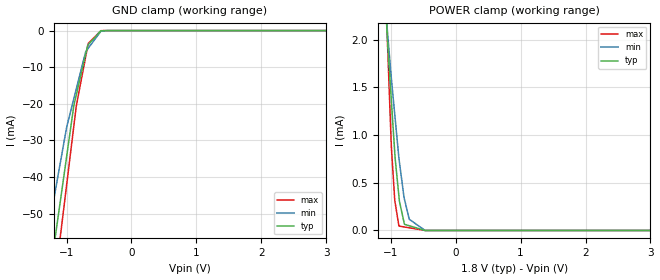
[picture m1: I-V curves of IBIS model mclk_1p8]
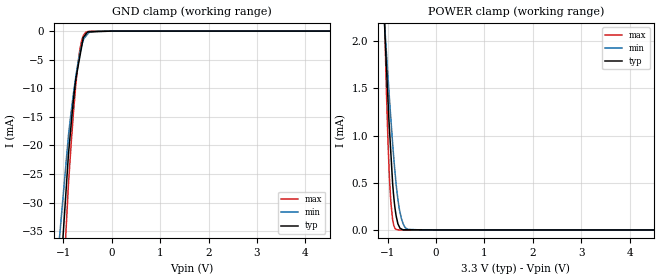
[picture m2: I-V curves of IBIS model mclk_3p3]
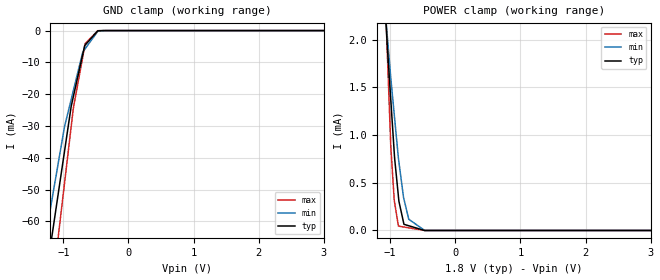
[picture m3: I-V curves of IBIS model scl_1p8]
|Texas Instruments Incorporated
| Low-Power Stereo Codec with 6 Inputs, 6 Outputs, Speaker/HP Amp and
| Enhanced Digital Effects
| Marketing part#   Digital Voltage Range   Package-type   #pins
| TLV320AIC3101IRHBR   1.1V - 3.6V   QFN   32
| TLV320AIC3101IRHBT   1.1V - 3.6V   QFN   32
| TLVAIC3101IRHBRG4   1.1V - 3.6V   QFN   32
| TLVAIC3101IRHBTG4   1.1V - 3.6V   QFN   32
[IBIS Ver]   4.1
[File name]   tlv320aic3101.ibs
[File Rev]   1.1
[Date]   10/26/2012
[Source]
| Texas Instruments Incorporated.
| Analog-eLab Design Center, HPA
| 12500 TI Blvd
| Dallas, TX -75243
| e-mail: elab_scm_ibis@list.ti.com
[Notes]   Revision History:
| Rev 1.1: 10/26/2012
| - Voltage range for modeling is changed for 3.3V models.
| Rev 1.0: 10/23/2012
| - Initial version of the model
| - Model generated from simulations in TISPICE
| - Model matched to SPICE simulation
| - C_comp although listed in numerical order of value are
|   obtained from varying PVT conditions. For PVT conditions for
|   each specific value refer the buffer description under
|   respective [Model]. IBIS model user is responsible for using
|   appropriate C_comp to simulate for Signal Integrity.
| - Model names with a trailing _1p8 contains the model for
|   1.8V [1.71V and 1.89V].Model names with a trailing _3p3
|   contains the model for 3.3V [2.7V and 3.6V].
| - The buffer characteristics for buffer on Pins (MCLK),
|   (DIN) and (_RESET) is same, hence replaced by a single model "mclk".
[Disclaimer]
| This model is designed as an aid for customers of Texas Instruments.
| TI and its licensors and suppliers make no warranties, either expressed
| or implied, with respect to this  model, including the warranties of
| merchantability or fitness for a particular purpose. The model is
| provided solely on an "as is" basis. The entire risk as to its quality
| and performance is with the customer.
[Copyright]
(C) Copyright 2012 Texas Instruments Incorporated.All rights reserved.
|   TLV320AIC3101
[Component]   TLV320AIC3101
[Manufacturer]   TI
[Package]   |32 QFN   -  RHB package
|   typ   min   max
R_pkg   0.07718   0.03258   0.11084
L_pkg   1.34741nH   0.76736nH   1.81874nH
C_pkg   0.19486pF   0.16263pF   0.25079pF
[Pin]  signal_name   model_name   R_pin   L_pin   C_pin
1   MCLK   MCLK   0.10980   1.80738nH  0.20351pF
2   BCLK   BW_CLK   0.04834   1.27894nH  0.25079pF
3   WCLK   BW_CLK   0.04153   1.05595nH  0.22423pF
4   DIN   MCLK   0.07341   1.17495nH  0.17505pF
5   DOUT   DOUT   0.06543   1.04328nH  0.16455pF
6   DVSS   GND   0.06617   1.05558nH  0.16473pF
7   IOVDD   POWER   0.07422   1.18976nH  0.17262pF
8   SCL   SCL   0.09445   1.54209nH  0.17632pF
9   SDA   SDA   0.10381   1.70349nH  0.18628pF
10   MIC1LP/LINE1LP   TERM   0.09706   1.57875nH  0.19190pF
11   MIC1LM/LINE1LM   TERM   0.11084   1.81874nH  0.21129pF
12   MIC1RP/LINE1RP   TERM   0.09921   1.61505nH  0.20474pF
13   MIC1RM/LINE1RM   TERM   0.09378   1.51996nH  0.19828pF
14   MIC2L/LINE2L/MICDET TERM   0.09457   1.53226nH  0.19911pF
15   MICBIAS   TERM   0.10123   1.64737nH  0.20366pF
16   MIC2R/LINE2R   TERM   0.11073   1.81870nH  0.19581pF
17   AVSS1   GND   0.10587   1.73309nH  0.18653pF
18   DRVDD   POWER   0.08549   1.37555nH  0.18063pF
19   HPLOUT   TERM   0.04394   1.15760nH  0.22090pF
20   HPLCOM   TERM   0.03761   0.93514nH  0.20874pF
21   DRVSS   GND   0.03475   0.83845nH  0.19402pF
22   HPRCOM   TERM   0.03258   0.76736nH  0.18547pF
23   HPROUT   TERM   0.03636   0.90542nH  0.19865pF
24   DRVDD   POWER   0.04412   1.17412nH  0.20375pF
25   AVDD   POWER   0.04645   1.25584nH  0.20175pF
26   AVSS2   GND   0.04847   1.29980nH  0.22244pF
27   LEFT_LOP   TERM   0.09345   1.51004nH  0.19823pF
28   LEFT_LOM   TERM   0.07850   1.25496nH  0.18383pF
29   RIGHT_LOP   TERM   0.06952   1.10594nH  0.17081pF
30   RIGHT_LOM   TERM   0.07016   1.11884nH  0.16699pF
31   _RESET   MCLK   0.06890   1.09832nH  0.16263pF
32   DVDD   POWER   0.10602   1.74027nH  0.18605pF
|   Model Selectors
[Model Selector] MCLK
mclk_1p8  1.8V digital input
mclk_3p3  3.3V digital input
[Model Selector] SCL
scl_1p8  1.8V digital input
scl_3p3  3.3V digital input
[Model Selector] DOUT
dout_1p8  1.8V digital 3-state
dout_3p3  3.3V digital 3-state
[Model Selector] BW_CLK
bw_clk_1p8  1.8V digital I/O
bw_clk_3p3  3.3V digital I/O
[Model Selector] SDA
sda_1p8  1.8V digital I/O Open Drain
sda_3p3  3.3V digital I/O Open Drain
[Model Selector] TERM
term_1-8V  1.8V nominal termination
term_3-3V  3.3V nominal termination
[Model] term_1-8V
Model_type Terminator
C_comp   1.0e-20F  1.0e-20F  1.0e-20F
|   typ   min   max
[Voltage Range]   1.8V   1.71V   1.89V
[POWER Clamp Reference]   1.8V   1.71V   1.89V
[GND Clamp Reference]   0V   0V   0V
|Ambient Temperature   25   85   -40
|Junction Temperature
[Temperature Range]   27   105   -40
[Model] term_3-3V
Model_type Terminator
C_comp   1.0e-20F  1.0e-20F  1.0e-20F
|   typ   min   max
[Voltage Range]   3.3V   2.7   3.6V
[POWER Clamp Reference]   3.3V   2.7   3.6V
[GND Clamp Reference]   0V   0V   0V
|Ambient Temperature   25   85   -40
|Junction Temperature
[Temperature Range]   27   105   -40
| Models and submodels in the file (12): mclk_1p8 (Input), mclk_3p3 (Input), scl_1p8 (Input), scl_3p3 (Input), dout_1p8 (3-state), dout_3p3 (3-state), bw_clk_1p8 (I/O), bw_clk_3p3 (I/O), sda_1p8 (I/O_open_drain), sda_3p3 (I/O_open_drain), term_1-8V (Terminator), term_3-3V (Terminator)
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|   mclk_1p8 Model
[Model]   mclk_1p8
Model_type   Input
Vinl = 0.54
Vinh = 1.26
|   typ   min   max
|   (nom PVT)   (fast PVT)   (slow PVT)
C_comp   1.043e-12   1.039e-12   1.043e-12
| Where nom  PVT is Nominal Process, 1.8V, 27C
|   Fast PVT is Strong Process,  1.89V, -40C
|   Slow PVT is Weak Process,   1.71V, 105C
[Model Spec]
|Subparameter   typ   min   max
Vinh   1.26   1.197   1.323
Vinl   0.54   0.513   0.567
[Voltage Range]   1.8   1.71   1.89
|Ambient Temperature   25   85   -40
|Junction Temperature
[Temperature Range]   27   105   -40
[Power Clamp Reference]   1.8   1.71   1.89
[GND Clamp Reference]   0   0   0
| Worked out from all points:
|   GND clamp passes 1 mA (typ) near -0.52 V on its own axis
|   POWER clamp passes 1 mA (typ) near -0.96 V on its own axis
[GND Clamp]
|   Voltage   I(typ)   I(min)   I(max)
-1.8V     -243.1mA   -121.9mA   -355.9mA
-1.51V    -98.55mA   -77.34mA   -126.4mA
-1.155V   -54.02mA   -41.99mA   -64.87mA
-996.9mV  -34.24mA   -26.29mA   -41.97mA
-885.6mV  -20.34mA   -18.46mA   -25.83mA
-848.6mV  -17.49mA   -15.86mA   -20.5mA
-704.5mV  -6.404mA   -5.754mA   -7.113mA
-673.2mV  -3.994mA   -5.009mA   -4.203mA
-665.3mV  -3.84mA    -4.821mA   -3.467mA
-470.6mV  -70.83uA   -188.8uA   -24.2uA
-287.3mV  -445.8nA   -2.215uA   -13.16nA
3.6V      0A         0A         0A
[POWER Clamp]
|   Voltage   I(typ)   I(min)   I(max)
-1.8V     11.74mA    8.633mA    19.35mA
-1.081V   2.386mA    2.338mA    2.535mA
-1.04V    1.89mA     2.005mA    1.793mA
-990.4mV  1.367mA    1.596mA    886.6uA
-937.4mV  814.2uA    1.215mA    315.3uA
-930.6mV  748.9uA    1.166mA    286.6uA
-873.2mV  356.4uA    756.1uA    45.76uA
-865.8mV  305.9uA    716.4uA    44.92uA
-788.4mV  64.55uA    328.2uA    36.12uA
-714.8mV  49.55uA    117.7uA    27.76uA
-470.3mV  0A         256.8nA    0A
3.6V      0A         0A         0A
|   mclk_3p3 Model
[Model]   mclk_3p3
Model_type   Input
Vinl = 0.99
Vinh = 2.31
|   typ   min   max
|   (nom PVT)   (fast PVT)   (slow PVT)
C_comp   9.787e-13   9.710e-13   9.903e-13
| Where nom  PVT is Nominal Process, 3.3V, 27C
|   Fast PVT is Strong Process,  3.6V, -40C
|   Slow PVT is Weak Process,   2.7V, 105C
[Model Spec]
|Subparameter   typ   min   max
Vinh   2.31   1.89   2.52
Vinl   0.99   0.81   1.08
[Voltage Range]   3.3   2.7   3.6
|Ambient Temperature   25   85   -40
|Junction Temperature
[Temperature Range]   27   105   -40
[Power Clamp Reference]   3.3   2.7   3.6
[GND Clamp Reference]   0   0   0
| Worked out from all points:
|   GND clamp passes 1 mA (typ) near -0.58 V on its own axis
|   POWER clamp passes 1 mA (typ) near -0.96 V on its own axis
[GND Clamp]
|   Voltage   I(typ)   I(min)   I(max)
-3.3V     -1.786A    -1.575A    -1.965A
-1.498V   -98.66mA   -76.19mA   -123.5mA
-897.6mV  -21.53mA   -18.27mA   -26.74mA
-842.4mV  -16.36mA   -14.17mA   -19.75mA
-772.2mV  -10.33mA   -9.522mA   -12.04mA
-745.8mV  -8.373mA   -7.959mA   -9.433mA
-702mV    -6.326mA   -5.63mA    -5.815mA
-622.8mV  -2.623mA   -2.458mA   -1.616mA
-590.7mV  -1.122mA   -1.587mA   -839.1uA
-532.8mV  -494.1uA   -836.1uA   -172.5uA
-286.2mV  -88.77uA   -2.151uA   -5.093uA
6.6V      0A         0A         0A
[POWER Clamp]
|   Voltage   I(typ)   I(min)   I(max)
-3.3V     32.15mA    22.38mA    56.05mA
-1.076V   2.305mA    2.283mA    2.475mA
-1.03V    1.766mA    1.906mA    1.532mA
-993.6mV  1.375mA    1.621mA    934uA
-964.8mV  1.081mA    1.4mA      561.5uA
-932.4mV  796.9uA    1.166mA    280.4uA
-881.1mV  387.7uA    807.4uA    64.82uA
-820.8mV  138.7uA    461.6uA    4.877uA
-766.8mV  41.34uA    246.3uA    409.3nA
-718.2mV  11.1uA     124.3uA    128.1nA
-583.2mV  2.076uA    6.133uA    0A
6.6V      0A         0A         0A
|   scl_1p8 Model
[Model]   scl_1p8
Model_type   Input
Vinl = 0.54
Vinh = 1.26
|   typ   min   max
|   (nom PVT)   (fast PVT)   (slow PVT)
C_comp   1.183e-12   1.183e-12   1.188e-12
| Where nom  PVT is Nominal Process, 1.8V, 27C
|   Fast PVT is Strong Process,  1.89V, -40C
|   Slow PVT is Weak Process,   1.71V, 105C
[Model Spec]
|Subparameter   typ   min   max
Vinh   1.26   1.197   1.323
Vinl   0.54   0.513   0.567
[Voltage Range]   1.8   1.71   1.89
|Ambient Temperature   25   85   -40
|Junction Temperature
[Temperature Range]   27   105   -40
[Power Clamp Reference]   1.8   1.71   1.89
[GND Clamp Reference]   0   0   0
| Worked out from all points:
|   GND clamp passes 1 mA (typ) near -0.51 V on its own axis
|   POWER clamp passes 1 mA (typ) near -0.96 V on its own axis
[GND Clamp]
|   Voltage   I(typ)   I(min)   I(max)
-1.8V     -260.7mA   -144.7mA   -374.8mA
-1.504V   -119.2mA   -92.4mA    -151.4mA
-1.177V   -65.03mA   -53.51mA   -83.53mA
-1.136V   -59.32mA   -48.6mA    -74.96mA
-983.2mV  -38.24mA   -30.45mA   -48.37mA
-878.4mV  -23.8mA    -21.63mA   -30.1mA
-844.8mV  -20.71mA   -18.82mA   -24.3mA
-701.1mV  -7.468mA   -6.764mA   -8.279mA
-671.4mV  -4.732mA   -5.922mA   -4.969mA
-663.4mV  -4.546mA   -5.695mA   -4.076mA
-470.6mV  -85.43uA   -227.6uA   -29.15uA
3.6V      0A         0A         0A
[POWER Clamp]
|   Voltage   I(typ)   I(min)   I(max)
-1.8V     11.74mA    8.633mA    19.35mA
-1.081V   2.386mA    2.338mA    2.535mA
-1.04V    1.89mA     2.005mA    1.793mA
-990.4mV  1.367mA    1.596mA    886.6uA
-937.4mV  814.2uA    1.215mA    315.3uA
-930.6mV  748.9uA    1.166mA    286.6uA
-873.2mV  356.4uA    756.1uA    45.76uA
-865.8mV  305.9uA    716.4uA    44.92uA
-788.4mV  64.55uA    328.2uA    36.12uA
-714.8mV  49.55uA    117.7uA    27.76uA
-470.3mV  0A         257nA      0A
3.6V      0A         0A         0A
